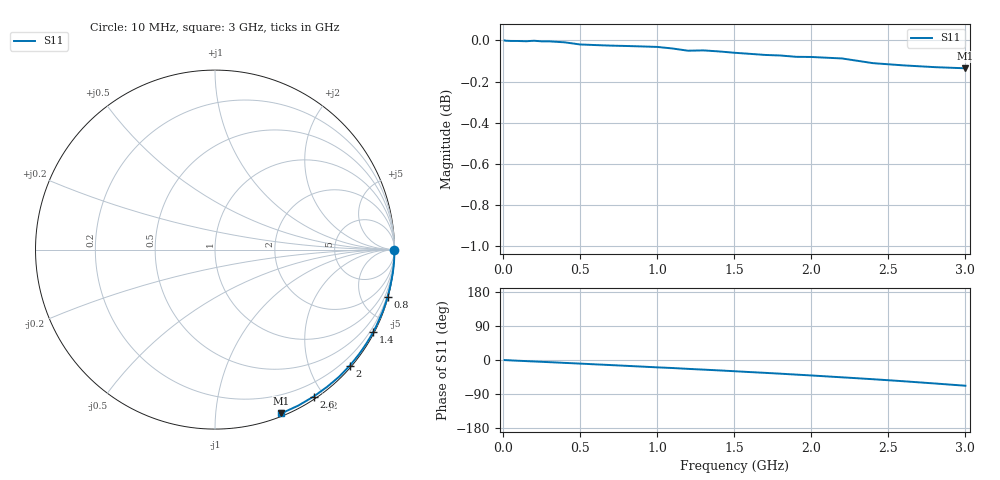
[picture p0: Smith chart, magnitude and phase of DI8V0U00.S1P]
! SIEMENS Small Signal Semiconductors
! BAV99
! Silicon Switching Diode in SOT23
! VR = 8 V
! S-Parameters:  May  1995
# GHz  S  MA  R  50
!  f  S11
! GHz  MAG  ANG
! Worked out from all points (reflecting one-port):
!   30 points, 10 MHz to 3 GHz, reference 50 ohm
!   lowest |S11| = -0.1 dB at 3 GHz (marker M1), VSWR 128.28, Z = 1.25 - j74.3 ohm
!   phase of S11 starts at -0 deg and turns -68 deg over the sweep
!   S11 on the Smith chart (normalised r, x): 10 MHz: open; 800 MHz: 0.09, -7.40; 1.4 GHz: 0.05, -4.10; 2 GHz: 0.04, -2.69; 2.6 GHz: 0.03, -1.88; 3 GHz: 0.02, -1.49
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0.01  1 -0.2
0.02  0.9998 -0.4
0.1  0.9997 -2.0
0.15  0.9995 -2.9
0.2  0.9998 -3.9
0.3  0.9995 -5.7
0.4  0.9989 -7.6
0.5  0.9978 -9.5
0.6  0.9974 -11.5
0.7  0.9971 -13.4
0.8  0.9969 -15.4
0.9  0.9967 -17.4
1  0.9964 -19.4
1.1  0.9955 -21.2
1.2  0.9943 -23.4
1.3  0.9944 -25.4
1.4  0.9939 -27.4
1.5  0.9931 -29.6
1.6  0.9925 -31.8
1.7  0.9919 -33.9
1.8  0.9916 -36.1
1.9  0.9909 -38.5
2  0.9908 -40.8
2.2  0.99 -45.7
2.4  0.9874 -50.7
2.6  0.9861 -56.1
2.8  0.9852 -61.9
3  0.9845 -67.9
